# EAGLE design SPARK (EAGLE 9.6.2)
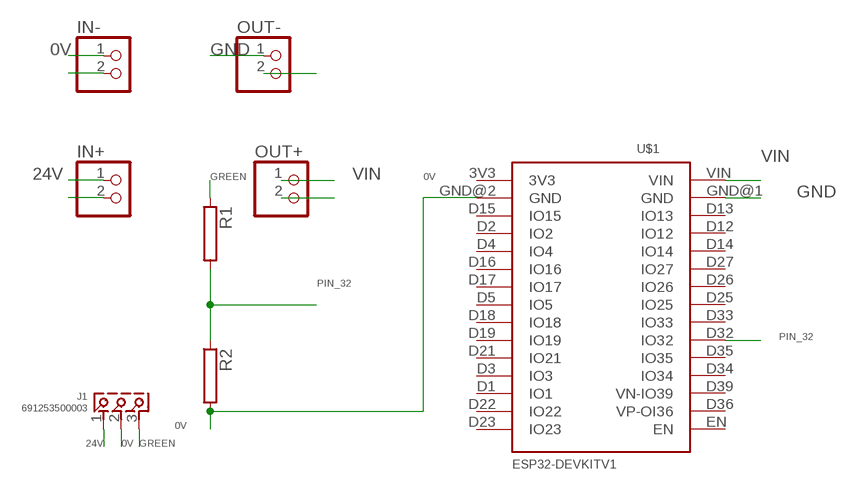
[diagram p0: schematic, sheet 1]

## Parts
IN+  PINHD-1X2  [1X02]
IN-  PINHD-1X2  [1X02]
J1  691253500003  [691253500003]
OUT+  PINHD-1X2  [1X02]
OUT-  PINHD-1X2  [1X02]
R1  RAC01  [AC01]
R2  RAC01  [AC01]
U$1  ESP32DEVKITV1  [ESP32-DEVKITV1]

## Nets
0V: IN-.1 J1.2 R2.2 U$1.GND@2(GND)
24V: IN+.1 J1.1
GND: OUT-.1 U$1.GND@1(GND)
GREEN: J1.3 R1.1
N$2: IN-.2
N$4: IN+.2
N$6: OUT-.2
N$8: OUT+.2
PIN_32: R1.2 R2.1 U$1.D32(IO32)
VIN: OUT+.1 U$1.VIN
Unconnected: U$1.3V3 U$1.D1(IO1) U$1.D2(IO2) U$1.D3(IO3) U$1.D4(IO4) U$1.D5(IO5) U$1.D12(IO12) U$1.D13(IO13) U$1.D14(IO14) U$1.D15(IO15) U$1.D16(IO16) U$1.D17(IO17) U$1.D18(IO18) U$1.D19(IO19) U$1.D21(IO21) U$1.D22(IO22) U$1.D23(IO23) U$1.D25(IO25) U$1.D26(IO26) U$1.D27(IO27) U$1.D33(IO33) U$1.D34(IO34) U$1.D35(IO35) U$1.D36(VP-OI36) U$1.D39(VN-IO39) U$1.EN

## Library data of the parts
IN+ IN- OUT+ OUT- = pinhead:PINHD-1X2: PIN HEADER
J1 = terminal block 3 pin:691253500003: WR-TBL Serie 2535 - 5.08 mm Vertical Entry Modular w. Rising Cage Clamp KIND PROPERTIES Pitch 5.08 mm MATERIAL PROPERTIES Insulator Material PA66 Insulator Flammability Rating UL94 V-0 Contact Material Copper Alloy Contact Plating Nickel Terminal Screw Material Steel Terminal Screw Plating Zinc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; AVAILABILITY: In Stock; CHECK_PRICES: https://www.snapeda.com/parts/691253500003/Wurth+Elektronik/view-part/?ref=eda; DESCRIPTION: 3 Position Wire to Board Terminal Block Vertical with Board 0.200 (5.08mm) Through Hole; MF: Würth Elektronik; MP: 691253500003; PACKAGE: None; PRICE: None; PURCHASE-URL: https://www.snapeda.com/api/url_track_click_mouser/?unipart_id=4503293&manufacturer=Würth Elektronik&part_name=691253500003&search_term=terminal block, 3 pin; SNAPEDA_LINK: https://www.snapeda.com/parts/691253500003/Wurth+Elektronik/view-part/?ref=snap
R1 R2 = resistor-power:R: Power Resitor; OC_FARNELL: unknown; OC_NEWARK: unknown
U$1 = ESP32-DEVKITV1:ESP32DEVKITV1

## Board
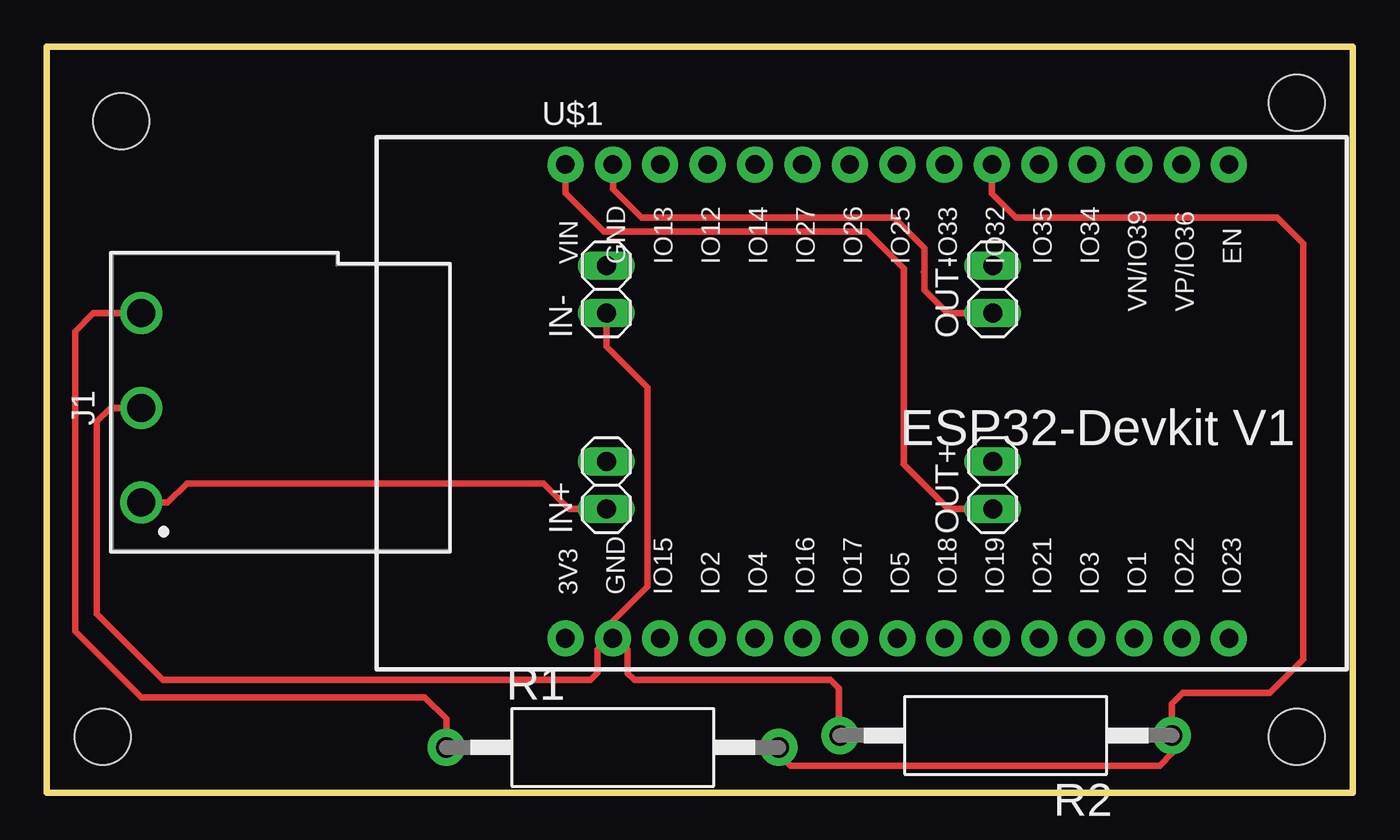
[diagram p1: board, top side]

Size 70 x 40 mm. Coordinates in mm from the lower left corner, seen from the top.
Outline: 0,0 70,0 70,40 0,40 0,0
Copper layers (1*16): Top 0.035mm / dielectric 1.5mm / Bottom 0.035mm
Design rules "default": minimum track width 6mil, minimum drill 0.35mm, track to track 6mil, track to pad 6mil, pad to pad 6mil, via to via 6mil, smd to smd 6mil, copper to edge 40mil, drill to drill 6mil, minimum pad ring 10mil, minimum via ring 8mil, stop-mask expansion 4mil, vias tented up to drill 0mil, thermal gap 10mil
Holes 3 mm at 4,36 3,3 67,37 67,3

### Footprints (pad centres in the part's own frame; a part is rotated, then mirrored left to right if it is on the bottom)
1X02 = drill 1.016 long: 1 -1.27,0; 2 1.27,0
691253500003 = drill 1.5: 1 -5.08,0; 2 0,0; 3 5.08,0
AC01 = drill 1.1 pad 2: 1 -8.9,0; 2 8.9,0
ESP32-DEVKITV1 = drill 1 pad 1.93: 3V3 -16.52,-12.27; D1 13.96,-12.27; D2 -8.9,-12.27; D3 11.42,-12.27; D4 -6.36,-12.27; D5 1.26,-12.27; D12 -8.9,13.135; D13 -11.44,13.135; D14 -6.36,13.135; D15 -11.44,-12.27; D16 -3.82,-12.27; D17 -1.28,-12.27; D18 3.8,-12.27; D19 6.34,-12.27; D21 8.88,-12.27; D22 16.5,-12.27; D23 19.04,-12.27; D25 1.26,13.135; D26 -1.28,13.135; D27 -3.82,13.135; D32 6.34,13.135; D33 3.8,13.135; D34 11.42,13.135; D35 8.88,13.135; D36 16.5,13.135; D39 13.96,13.135; EN 19.04,13.135; GND@1 -13.98,13.135; GND@2 -13.98,-12.27; VIN -16.52,13.135

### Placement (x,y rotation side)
IN+  30,16.5 90 top
IN-  30,27 90 top
J1  5.08,20.64 90 top
OUT+  50.7,16.5 90 top
OUT-  50.7,27 90 top
R1  30.33,2.44 0 top
R2  51.41,3.07 180 top
U$1  44.32,20.55 0 top

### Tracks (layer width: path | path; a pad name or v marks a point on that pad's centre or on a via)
0V
  Top 0.34: J1.2 3.43,20.64 2.69,19.9 2.69,9.6 6.22,6.07 29.16,6.07 29.52,6.43 29.52,7.68 30.11,8.28 U$1.GND@2 | R2.2 42.46,3.12 42.46,5.6 42.01,6.04 31.5,6.04 31.14,6.4 31.14,7.68 30.55,8.28 U$1.GND@2 | IN-.1 30,23.93 32.2,21.72 32.2,11.07 30.34,9.21 U$1.GND@2
24V
  Top 0.34: J1.1 6.49,15.56 7.52,16.59 26.64,16.59 27.99,15.23 IN+.1
GND
  Top 0.34: U$1.GND@1 30.34,32.37 31.88,30.84 45.41,30.84 47.04,29.21 47.04,27.89 | OUT-.1 48.26,25.73 47.04,26.95 47.04,27.89 | 47.04,27.89 47.02,27.91
GREEN
  Top 0.34: R1.1 21.43,3.96 20.26,5.13 5.05,5.13 1.52,8.66 1.52,24.74 2.5,25.72 J1.3
PIN_32
  Top 0.34: R1.2 39.23,2.08 39.86,1.45 59.65,1.45 60.31,2.11 R2.1 60.31,4.78 60.89,5.36 65.54,5.36 67.33,7.15 67.33,29.44 65.94,30.84 51.94,30.84 50.66,32.11 U$1.D32
VIN
  Top 0.34: U$1.VIN 27.8,32.14 29.87,30.07 43.97,30.07 45.94,28.11 45.94,17.61 | OUT+.1 48.32,15.23 45.94,17.61 | 45.92,17.63 45.94,17.61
